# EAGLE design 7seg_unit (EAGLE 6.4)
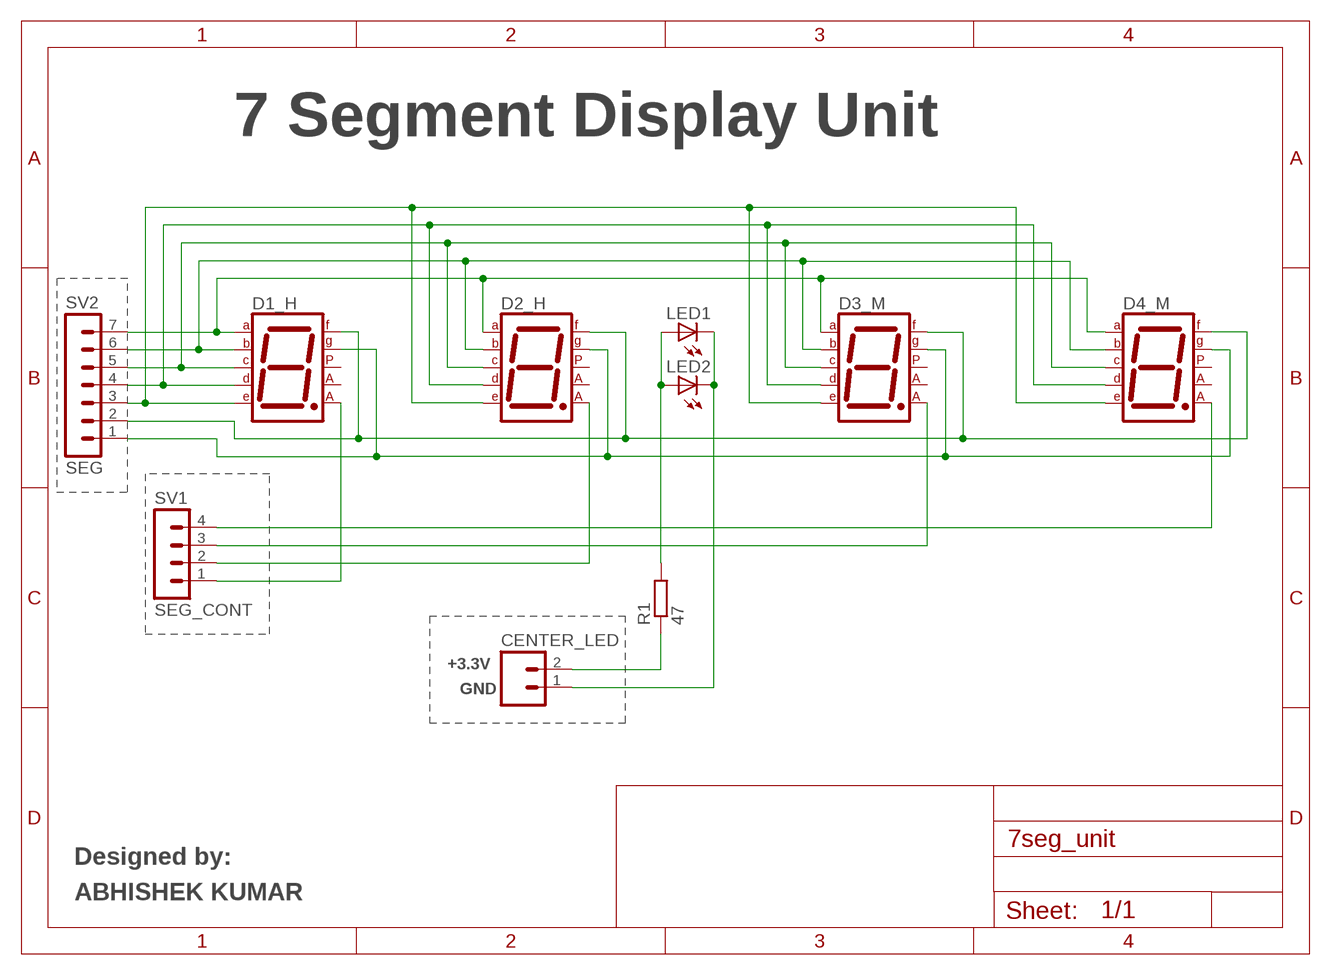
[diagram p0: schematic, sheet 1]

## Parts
CENTER_LED  M02LOCK  [1X02_LOCK]
D1_H  7SEG-CA  [7SEG-13]
D2_H  7SEG-CA  [7SEG-13]
D3_M  7SEG-CA  [7SEG-13]
D4_M  7SEG-CA  [7SEG-13]
LED1  LED3MM  [LED3MM]
LED2  LED3MM  [LED3MM]
R1  47  R-EU_M1206  [M1206]
SV1  SEG_CONT  MA04-1  [MA04-1]
SV2  SEG  MA07-1  [MA07-1]

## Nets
N$1: D1_H.1(E) D2_H.1(E) D3_M.1(E) D4_M.1(E) SV2.3
N$2: D1_H.2(D) D2_H.2(D) D3_M.2(D) D4_M.2(D) SV2.4
N$3: D1_H.4(C) D2_H.4(C) D3_M.4(C) D4_M.4(C) SV2.5
N$4: D1_H.6(B) D2_H.6(B) D3_M.6(B) D4_M.6(B) SV2.6
N$5: D1_H.7(A) D2_H.7(A) D3_M.7(A) D4_M.7(A) SV2.7
N$6: D1_H.9(F) D2_H.9(F) D3_M.9(F) D4_M.9(F) SV2.2
N$7: D1_H.10(G) D2_H.10(G) D3_M.10(G) D4_M.10(G) SV2.1
N$8: D4_M.8(CA2) SV1.4
N$9: D3_M.8(CA2) SV1.3
N$10: D2_H.8(CA2) SV1.2
N$11: D1_H.8(CA2) SV1.1
N$12: CENTER_LED.2 R1.1
N$13: CENTER_LED.1 LED1.K(C) LED2.K(C)
N$14: LED1.A LED2.A R1.2
Unconnected: D1_H.3(CA1) D1_H.5(DP) D2_H.3(CA1) D2_H.5(DP) D3_M.3(CA1) D3_M.5(DP) D4_M.3(CA1) D4_M.5(DP)

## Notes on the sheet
- 7 Segment Display Unit
- +3.3V
- GND
- Designed by:
- ABHISHEK KUMAR

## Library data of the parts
CENTER_LED = SparkFun:M02: Header 2
D1_H D2_H D3_M D4_M = special:7SEG-CA: 7-segment DISPLAY single anode, 13 mm
LED1 LED2 = led:LED: LED
R1 = resistor:R-EU_: RESISTOR, European symbol
SV1 = con-lstb:MA04-1: PIN HEADER; OC_FARNELL: unknown; OC_NEWARK: unknown
SV2 = con-lstb:MA07-1: PIN HEADER; OC_FARNELL: unknown; OC_NEWARK: unknown

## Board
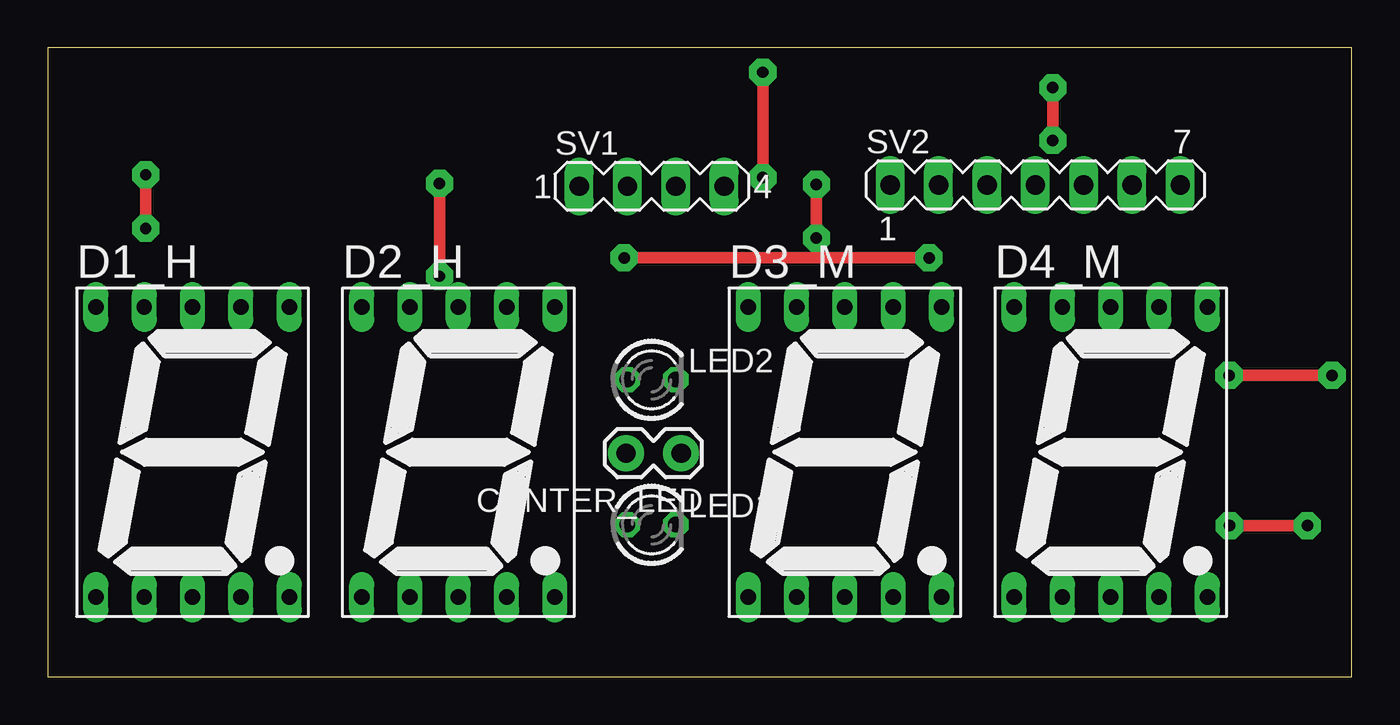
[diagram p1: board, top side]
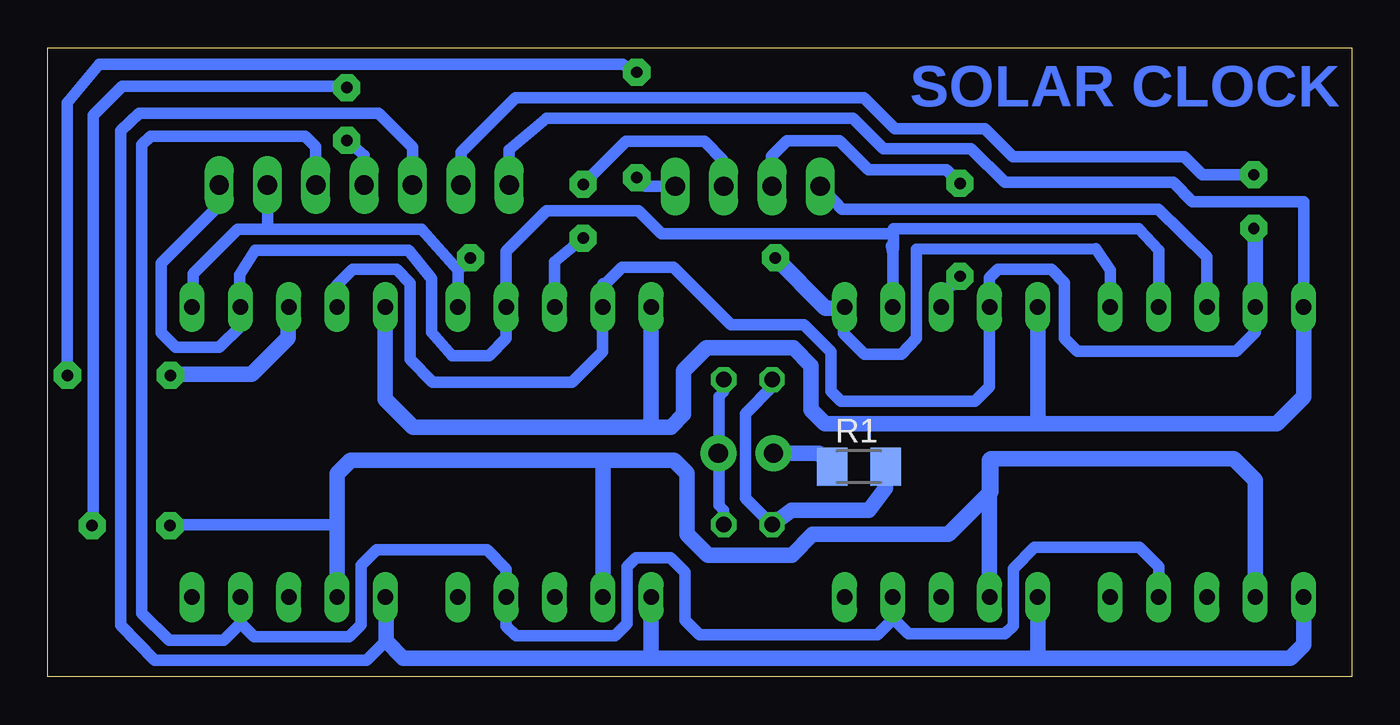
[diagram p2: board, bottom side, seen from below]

Size 68.56 x 33.07 mm. Coordinates in mm from the lower left corner, seen from the top.
Outline: 0,0 68.56,0 68.56,33.07 0,33.07 0,0
Copper layers (1*16): Top 0.035mm / dielectric 1.5mm / Bottom 0.035mm
Design rules "default": minimum track width 10mil, minimum drill 24mil, track to track 8mil, track to pad 8mil, pad to pad 8mil, via to via 8mil, smd to smd 8mil, copper to edge 40mil, drill to drill 8mil, minimum pad ring 10mil, minimum via ring 8mil, stop-mask expansion 4mil, vias tented up to drill 0mil, thermal gap 10mil

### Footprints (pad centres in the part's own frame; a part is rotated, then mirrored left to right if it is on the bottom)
1X02_LOCK = drill 1.016 pad 1.88: 1 -0.178,0; 2 2.718,0
7SEG-13 = drill 0.813 long: 1 -5.08,-7.62; 2 -2.54,-7.62; 3 0,-7.62; 4 2.54,-7.62; 5 5.08,-7.62; 6 5.08,7.62; 7 2.54,7.62; 8 0,7.62; 9 -2.54,7.62; 10 -5.08,7.62
LED3MM = drill 0.813 octagon: A -1.27,0; K 1.27,0
M1206 = smd 1.6 x 2: 1 -1.4,0; 2 1.4,0
MA04-1 = drill 1.016 long: 1 -3.81,0; 2 -1.27,0; 3 1.27,0; 4 3.81,0
MA07-1 = drill 1.016 long: 1 -7.62,0; 2 -5.08,0; 3 -2.54,0; 4 0,0; 5 2.54,0; 6 5.08,0; 7 7.62,0

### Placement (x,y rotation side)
CENTER_LED  33.12,11.76 180 top
D1_H  7.62,11.81 0 top
D2_H  21.59,11.81 0 top
D3_M  41.91,11.81 0 top
D4_M  55.88,11.81 0 top
LED1  31.75,8 0 top
LED2  31.75,15.62 0 top
R1  25.91,11.05 0 bottom
SV1  31.75,25.78 0 top
SV2  51.92,25.86 0 top

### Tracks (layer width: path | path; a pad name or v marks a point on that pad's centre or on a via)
N$1
  Bottom 0.61: SV2.3 49.38,27.84 51.16,29.62 63.75,29.62 64.72,28.7 64.72,2.72 62.94,0.89 51.79,0.89 50.77,1.9
  Bottom 0.813: D1_H.1 2.54,1.7 3.25,0.99 16.51,0.99 | 16.51,0.99 37.03,0.99 | 37.03,0.99 49.86,0.99 50.77,1.9 50.77,4.17 D4_M.1 | D3_M.1 36.83,1.19 37.03,0.99 | D2_H.1 16.51,0.99
N$2  (via drill 0.6 pad 1.42)
  Top 0.61: v52.83,28.19 v52.83,30.96 | v66.22,7.95 v62.13,7.95
  Bottom 0.61: SV2.4 51.92,27.41 v52.83,28.19 | v52.83,30.96 53.34,31.04 64.64,31.04 66.17,29.51 66.17,8.05 v66.22,7.95 | v62.13,7.95 61.7,8 53.34,8
  Bottom 0.813: D1_H.2 5.08,10.34 6.2,11.45 18.97,11.45 | 39.42,11.38 35.64,11.38 34.95,10.69 34.95,7.49 33.86,6.4 29.44,6.4 28.35,7.49 21.21,7.49 18.97,9.73 18.97,11.45 | 39.42,11.38 52.63,11.38 53.34,10.67 53.34,8 D4_M.2 | D3_M.2 39.37,11.33 39.42,11.38 | D2_H.2 19.05,11.38 18.97,11.45
N$3
  Bottom 0.61: D1_H.4 10.16,5.79 11.18,6.81 16.69,6.81 17.8,5.69 17.8,2.69 18.24,2.26 23.32,2.26 24.13,3.07 D2_H.4 24.13,3.02 24.94,2.21 34.29,2.21 35.05,2.97 35.05,5.51 35.81,6.27 37.62,6.27 38.1,5.79 38.1,2.79 38.73,2.16 43.94,2.16 44.45,2.67 D3_M.4 44.45,5.66 45.47,6.68 51.26,6.68 52.07,5.87 52.07,2.74 52.71,2.11 57.71,2.11 58.42,2.82 | 58.42,2.82 D4_M.4 | SV2.5 54.46,27.86 55.02,28.42 63.14,28.42 63.6,27.96 63.6,3.35 62.18,1.93 59.31,1.93 58.42,2.82
N$4  (via drill 0.6 pad 1.42)
  Top 0.61: v30.3,22.02 v46.33,22.02
  Bottom 0.61: D1_H.6 12.7,21.36 13.46,22.5 22.88,22.48 22.88,17.8 23.67,16.97 25.63,16.97 26.72,18.06 26.72,19.38 D2_H.6 | D4_M.6 60.96,20.52 60.91,20.57 60.91,21.18 58.57,23.52 57.02,23.52 | 57.02,23.52 48.9,23.52 46.99,21.36 | 46.99,21.36 D3_M.6 | SV2.6 57,23.55 57.02,23.52 | v46.33,22.02 46.99,21.36
  Bottom 0.813: 26.72,19.38 27.66,19.38 v30.3,22.02
N$5
  Bottom 0.61: D1_H.7 10.16,22.43 11.2,23.55 24.1,23.55 24.1,23.37 | 24.1,23.37 24.1,22.58 24.13,22.28 | 24.13,22.28 D2_H.7 | 24.21,22.66 24.13,22.28 | SV2.7 59.54,24.79 62.59,21.74 62.59,18.08 61.82,17.32 59.54,17.32 58.42,18.44 D4_M.7 58.47,19.48 58.47,21.13 57.66,22.43 49.58,22.43 48.39,20.93 48.39,18.11 47.29,16.89 45.36,16.89 44.45,17.8 D3_M.7 44.45,22.38 42.34,24.49 37.49,24.49 36.3,23.29 24.18,23.29 24.1,23.37
N$6  (via drill 0.6 pad 1.42)
  Top 0.61: v5.16,26.39 v5.16,23.57
  Bottom 0.61: D1_H.9 5.08,18.11 6.07,17.12 14.43,17.12 15.11,17.8 15.11,20.73 15.8,21.41 18.62,21.41 19.05,20.98 D2_H.9 19.05,15.24 19.81,14.48 26.85,14.48 27.38,15.01 27.38,17.09 28.8,18.52 32.64,18.52 35.66,21.54 38.35,21.54 39.37,20.52 | 39.37,20.52 D3_M.9 39.4,19.41 39.4,17.09 41,15.49 48.31,15.49 49.51,16.69 49.51,20.7 50.22,21.41 52.53,21.41 53.37,20.57 53.37,19.46 D4_M.9 | 39.37,20.52 39.37,20.65 | SV2.2 46.84,27.56 43.97,30.43 25.65,30.43 24.03,28.8 19.3,28.8 17.83,27.33 8.81,27.33 7.87,26.39 v5.16,26.39 | v5.16,23.57 5.08,23.06
  Bottom 0.813: 5.08,23.06 D1_H.9
N$7
  Bottom 0.61: SV2.1 44.3,27.71 42.37,29.34 42.34,29.36 26.24,29.36 24.64,27.76 20.02,27.76 18.24,25.98 9.4,25.98 8.38,24.97 2.54,24.97 D1_H.10
  Bottom 0.813: D1_H.10 2.54,14.73 3.96,13.31 16.26,13.31 | 16.26,13.31 27.69,13.31 28.42,14.05 28.42,16.36 29.36,17.3 33.93,17.3 35.13,16.1 35.13,13.79 35.79,13.13 37.11,13.13 | 37.11,13.13 49.35,13.13 50.82,14.6 50.82,19.41 D4_M.10 | D2_H.10 16.51,13.56 16.26,13.31 | D3_M.10 36.83,13.41 37.11,13.13
N$8  (via drill 0.6 pad 1.42)
  Top 0.61: v37.59,26.24 v37.59,31.77 | v67.51,15.85 v62.1,15.85
  Bottom 0.61: SV1.4 37.13,25.78 v37.59,26.24 | v37.59,31.77 38.33,32.21 65.84,32.21 67.54,30.17 67.54,15.8 v67.51,15.85 | v62.1,15.85 62.18,15.9 | 55.9,19.41 D4_M.8
  Bottom 0.813: 62.18,15.9 57.84,15.9 55.9,17.83 55.9,19.41
N$9  (via drill 0.6 pad 1.42)
  Top 0.61: v40.41,23.06 v40.41,25.88
  Bottom 0.61: D3_M.8 41.91,21.82 v40.41,23.06 | v40.41,25.88 38.15,28.14 34.04,28.14 33.05,27.15 33.05,25.81 SV1.3
N$10  (via drill 0.6 pad 1.42)
  Top 0.61: v20.6,21.06 v20.6,25.93
  Bottom 0.61: D2_H.8 21.59,20.07 v20.6,21.06 | v20.6,25.93 21.31,26.64 25.42,26.64 26.95,28.17 29.69,28.17 30.51,27.36 30.51,25.81 SV1.2
N$11
  Bottom 0.61: D1_H.8 7.62,22.07 10.18,24.59 26.8,24.59 SV1.1
N$12
  Bottom 0.813: CENTER_LED.2 28.02,11.76 R1.1
  Bottom 1.016: 30.48,11.84 CENTER_LED.2 30.48,11.68
N$13
  Bottom 0.61: LED1.K 33.02,8.76 33.27,9.02 33.27,11.73 CENTER_LED.1 33.27,11.79 33.27,14.73 33.02,14.99 LED2.K
N$14
  Bottom 0.61: LED2.A 30.48,15.24 31.88,13.84 31.88,9.4 LED1.A
  Bottom 0.813: R1.2 24.51,9.91 25.4,8.76 29.46,8.76 LED1.A

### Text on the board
Bottom: SOLAR CLOCK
